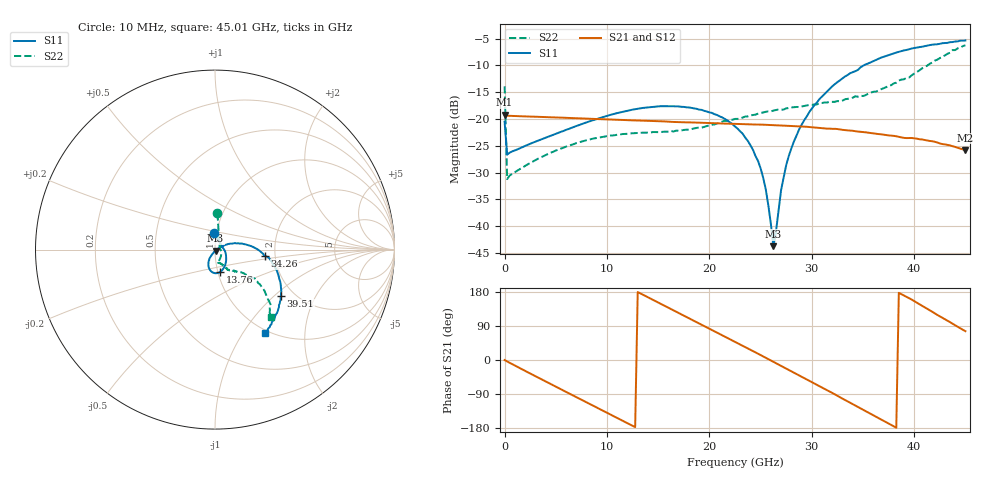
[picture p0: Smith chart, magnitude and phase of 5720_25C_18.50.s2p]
! Device:  ADRF5720
! Description: 0.5dB LSB GaAs MMIC 6-bit Digital Attenuator
! Frequency:  0.000009 -  40 GHz
! Ports:
!	RF1	= Port 1
!	RF2	= Port 2
! Vdd:  3.3 Volt
! Vss:  -3.3 Volt
! Control:  0/3.3 Volt
! State:  18.50 dB attenuation
! Data:  The device was measured using G-S-G Probes on a matrix board.
!  Data was collected using an calibrated 4 port network analyzer.
!  The reference plane for this measurement is at the launchers.
! Note:  Analog Devices supplies this data as a sample of measured data
!  for this product.  Your particular data for this product may vary.
!  Data was taken at 25 degrees C.
!  Analog Devices reserves the right to change this data at anytime.
# GHZ S DB R 45.0
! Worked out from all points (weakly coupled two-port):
!   181 points, 10 MHz to 45.01 GHz, reference 45 ohm
!   highest |S21| = -19.20 dB at 10 MHz (marker M1); lowest = -25.8 dB at 45.01 GHz (marker M2)
!   lowest |S11| = -43.7 dB at 26.26 GHz (marker M3), VSWR 1.01, Z = 45.3 - j0.508 ohm
!   |S11| at or under -10 dB: start of sweep to 35.08 GHz
!   |S22| runs from -31.2 to -6.2 dB; largest |S21 - S12| = 0.00016
!   S11 on the Smith chart (normalised r, x): 10 MHz: 0.97, +0.18; 13.76 GHz: 1.03, -0.26; 34.26 GHz: 1.76, -0.14; 39.51 GHz: 1.72, -1.10; 45.01 GHz: 0.96, -1.26
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0.01  -20.52 94.9  -19.20 -0.1  -19.20 -0.1  -13.89 86.1
0.26  -26.64 10.4  -19.39 -3.9  -19.39 -3.9  -31.21 16.8
3.26  -24.05 -18.8  -19.59 -46.1  -19.59 -46.1  -27.42 -33.9
7.76  -20.79 -48.0  -19.90 -108.3  -19.90 -108.3  -24.08 -66.7
13.76  -17.88 -77.0  -20.33 169.0  -20.33 169.0  -22.56 -78.5
15.26  -17.61 -83.6  -20.42 148.1  -20.42 148.1  -22.41 -77.5
19.26  -18.30 -101.2  -20.70 92.9  -20.70 92.9  -21.61 -68.4
22.76  -21.79 -116.9  -20.93 44.4  -20.93 44.4  -19.98 -61.5
24.01  -24.87 -121.7  -21.02 27.0  -21.02 27.1  -19.33 -60.4
25.01  -29.20 -121.8  -21.04 13.0  -21.05 13.1  -18.85 -59.8
25.51  -33.08 -116.5  -21.08 5.9  -21.08 5.9  -18.65 -60.1
26.26  -43.73 -59.5  -21.14 -4.7  -21.14 -4.7  -18.43 -58.0
26.51  -41.03 -10.6  -21.16 -8.2  -21.16 -8.2  -18.33 -59.5
27.01  -33.27 19.0  -21.19 -15.3  -21.19 -15.3  -18.26 -58.7
27.76  -26.92 26.3  -21.28 -26.0  -21.28 -26.0  -17.95 -58.0
28.76  -21.99 22.9  -21.37 -40.2  -21.37 -40.2  -17.76 -57.9
30.26  -17.44 15.3  -21.57 -62.0  -21.57 -61.9  -17.27 -56.1
32.26  -13.49 4.2  -21.83 -90.5  -21.84 -90.5  -16.79 -52.8
34.26  -11.07 -7.3  -22.27 -120.1  -22.26 -120.1  -15.76 -48.1
37.76  -7.90 -25.9  -23.09 -171.1  -23.09 -171.1  -13.69 -39.4
39.51  -6.97 -34.8  -23.56 163.4  -23.57 163.4  -12.26 -38.4
45.01  -5.34 -59.3  -25.80 76.1  -25.80 76.1  -6.23 -50.3
